(* Logix 5000 AddOnInstructionDefinition export Motor_Conv; software revision 20.01 *)

TYPE Motor_Conv_Type :   // Conveyor data
STRUCT
   Run_Status : BOOL;   // Run Status (1=running)
   Any_Fail : BOOL;   // Overall Failure Alarm (1= alarm)
   Aux_Fail : BOOL;   // Auxiliary failure alarm (1=alarm)
   SS_Fail : BOOL;   // Speed Switch failure alarm (1=alarm)
   OL_Fail : BOOL;   // Overload alarm (1=alarm)
   HOA_Fail : BOOL;   // HOA-switch-not-in-auto alarm (1-alarm)
   Seq_Start : BOOL;   // Motor start initiated from sequence
   Seq_Stop : BOOL;   // Motor stop initiated from sequence
END_STRUCT
END_TYPE

ADD_ON_INSTRUCTION Motor_Conv   (* revision 1.3 *)
// Conveyor motor control
VAR_INPUT
   Aux_Contact : BOOL; {required}   // Auxillary contact physical input
   OL_Trip : BOOL; {required}   // Overload trip contact physical input
   HOA_Switch : BOOL; {required}   // Hand-Off-Auto switch contact physical input (on when in Auto position)
   Speed_Switch : BOOL; {required}   // Speed Switch physical input (1=running)
   Alarm_Reset : BOOL; {required}   // Resets alarms
   Maint : BOOL; {required}   // Unit Maintenance/Operate Privilege
   Man_Start : BOOL; {required}   // Manual start for unit
   Man_Stop : BOOL; {required}   // Manual stop for unit
   Select_Dev_Num : DINT; {required}   // Number of device started/stopped at OI
   This_Dev_Num : DINT; {required}   // Number of this device for OI control
END_VAR
VAR_OUTPUT
   Starter : BOOL; {access Read Only, required}   // Motor starter contact physical input
END_VAR
VAR_IN_OUT
   Tag : Motor_Conv_Type; {required}   // Motor Tag
END_VAR
VAR
   Start_Req : BOOL;   // Internal used for start logic
   Stop_Req : BOOL;   // Internal used for stop logic
   Fail_Tmr : TIMER := (PRE := 40000);   // Timer for aux-fail alarm
   SS_Fail_Tmr : TIMER := (PRE := 20000);   // Timer for Speed switch fail alarm
END_VAR

ROUTINE Logic   (* ladder *)
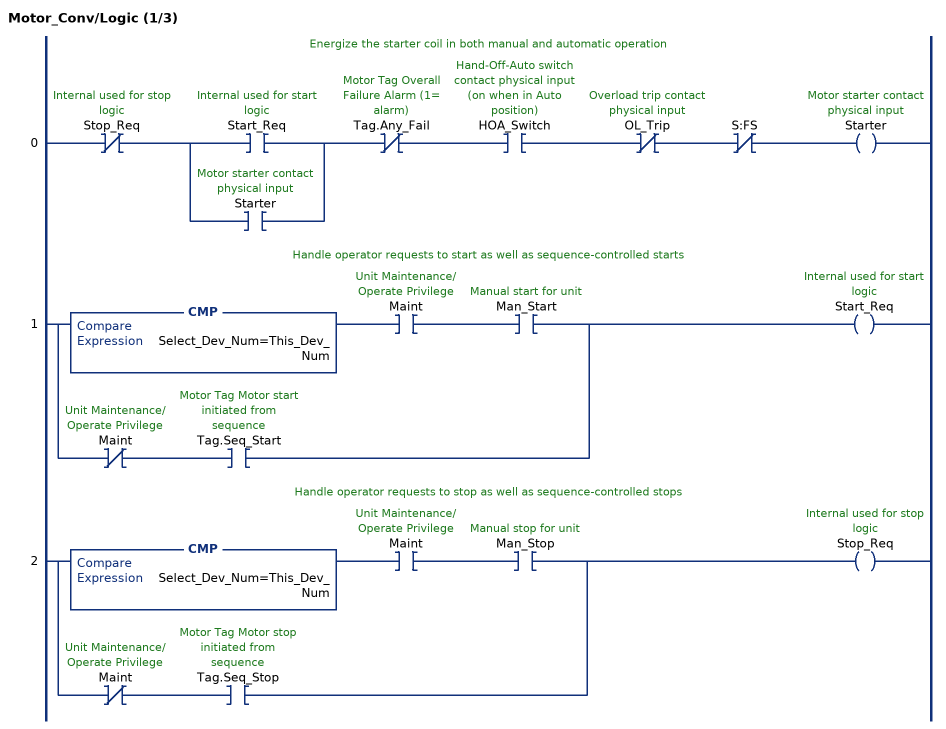
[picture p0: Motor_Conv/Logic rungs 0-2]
   // Energize the starter coil in both manual and automatic operation
   0: XIO(Stop_Req)[XIC(Start_Req) ,XIC(Starter) ]XIO(Tag.Any_Fail)XIC(HOA_Switch)XIO(OL_Trip)XIO(S:FS)OTE(Starter);
   // Handle operator requests to start as well as sequence-controlled starts
   1: [CMP(Select_Dev_Num=This_Dev_Num) XIC(Maint) XIC(Man_Start) ,XIO(Maint) XIC(Tag.Seq_Start) ]OTE(Start_Req);
   // Handle operator requests to stop as well as sequence-controlled stops
   2: [CMP(Select_Dev_Num=This_Dev_Num) XIC(Maint) XIC(Man_Stop) ,XIO(Maint) XIC(Tag.Seq_Stop) ]OTE(Stop_Req);
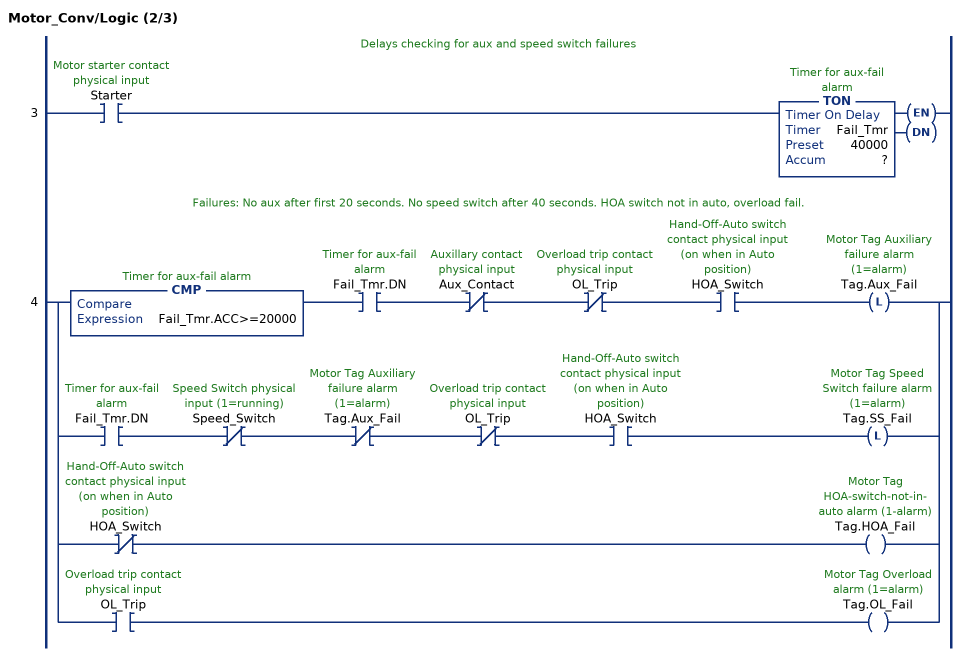
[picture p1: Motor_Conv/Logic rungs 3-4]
   // Delays checking for aux and speed switch failures
   3: XIC(Starter)TON(Fail_Tmr,?,?);
   // Failures: No aux after first 20 seconds. No speed switch after 40 seconds. HOA switch not in auto, overload fail.
   4: [CMP(Fail_Tmr.ACC>=20000) XIC(Fail_Tmr.DN) XIO(Aux_Contact) XIO(OL_Trip) XIC(HOA_Switch) OTL(Tag.Aux_Fail) ,XIC(Fail_Tmr.DN) XIO(Speed_Switch) XIO(Tag.Aux_Fail) XIO(OL_Trip) XIC(HOA_Switch) OTL(Tag.SS_Fail) ,XIO(HOA_Switch) OTE(Tag.HOA_Fail) ,XIC(OL_Trip) OTE(Tag.OL_Fail) ];
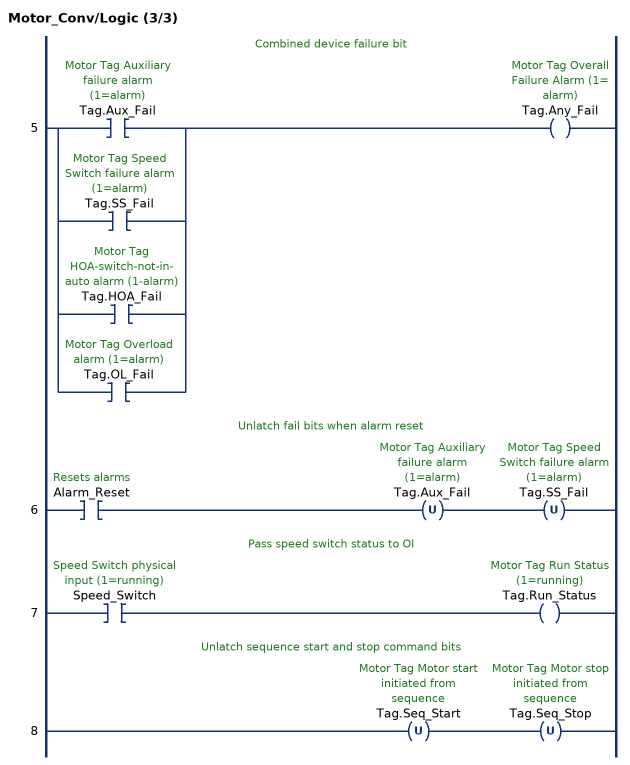
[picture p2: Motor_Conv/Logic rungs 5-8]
   // Combined device failure bit
   5: [XIC(Tag.Aux_Fail) ,XIC(Tag.SS_Fail) ,XIC(Tag.HOA_Fail) ,XIC(Tag.OL_Fail) ]OTE(Tag.Any_Fail);
   // Unlatch fail bits when alarm reset
   6: XIC(Alarm_Reset)OTU(Tag.Aux_Fail)OTU(Tag.SS_Fail);
   // Pass speed switch status to OI
   7: XIC(Speed_Switch)OTE(Tag.Run_Status);
   // Unlatch sequence start and stop command bits
   8: OTU(Tag.Seq_Start)OTU(Tag.Seq_Stop);
END_ROUTINE
END_ADD_ON_INSTRUCTION
